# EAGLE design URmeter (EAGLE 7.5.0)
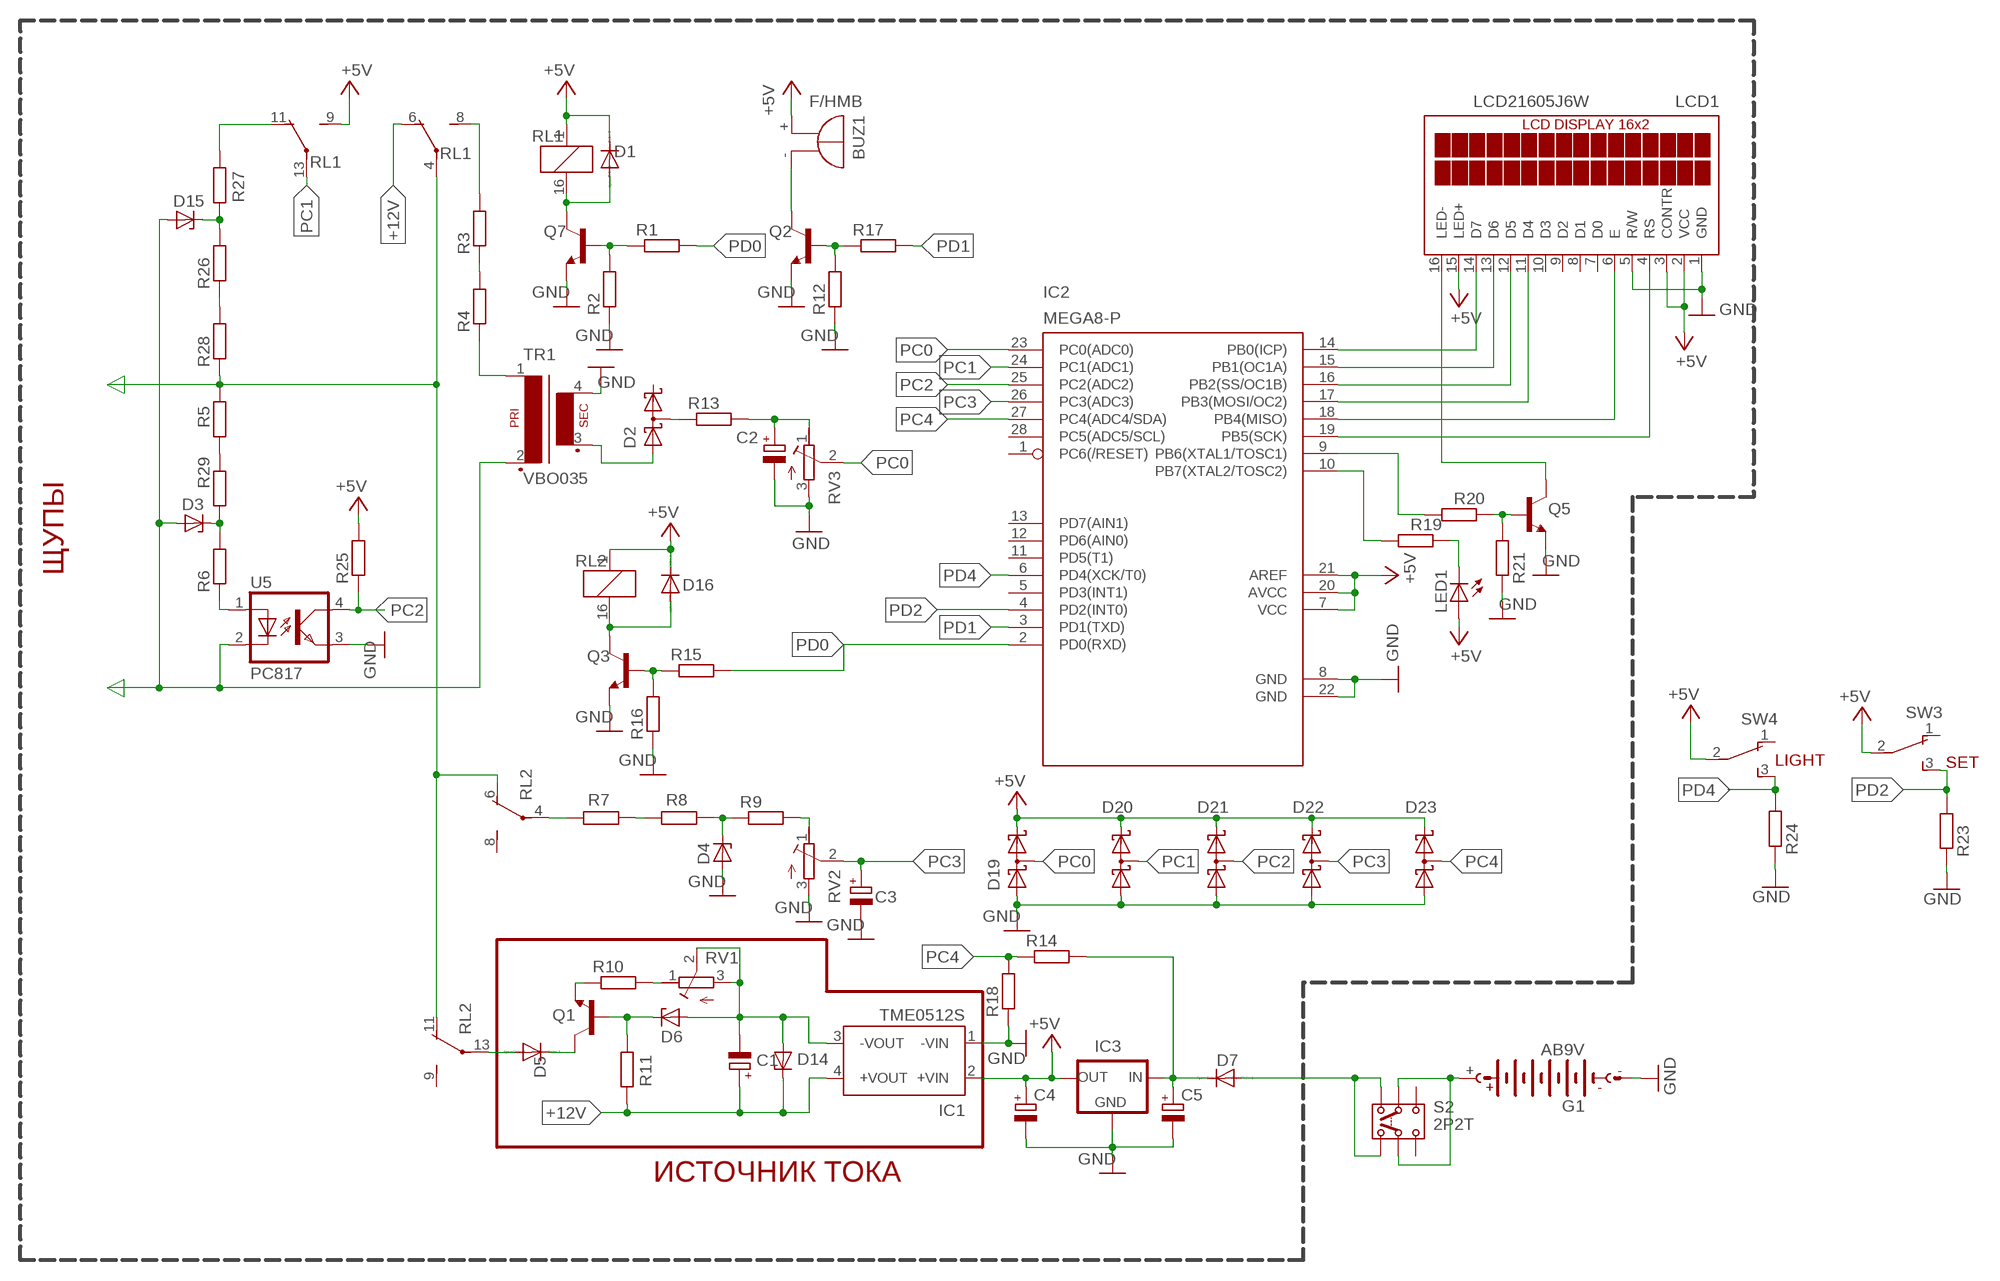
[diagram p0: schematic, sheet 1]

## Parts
BUZ1  F/HMB  [F/HMB]
C1  CPOL-EUE2-5  [E2-5]
C2  CPOL-EUE2-5  [E2-5]
C3  CPOL-EUE2-5  [E2-5]
C4  CPOL-EUE2-5  [E2-5]
C5  CPOL-EUE2-5  [E2-5]
D1  CGRM4007-G  [SOD-123_MINI-SMA]
D2  BAT54S  [SOT23]
D3  BZX85  [DO41Z10]
D4  BZX85  [DO41Z10]
D5  CGRM4007-G  [SOD-123_MINI-SMA]
D6  BZX85  [DO41Z10]
D7  CGRM4007-G  [SOD-123_MINI-SMA]
D14  BZX85  [DO41Z10]
D15  BZX85  [DO41Z10]
D16  CGRM4007-G  [SOD-123_MINI-SMA]
D19  BAT54S  [SOT23]
D20  BAT54S  [SOT23]
D21  BAT54S  [SOT23]
D22  BAT54S  [SOT23]
D23  BAT54S  [SOT23]
G1  AB9V  [AB9V]
IC1  TME0512S  [TME]
IC2  MEGA8-P  [DIL28-3]
IC3  78XXL  [78XXL]
LCD1  LCD21605J6W  [LCD21605J6W]
LED1  LED3MM  [LED3MM]
Q1  KSC5026MOS  -NPN-TO126  [TO126]
Q2  BC847  [SOT23]
Q3  BC847  [SOT23]
Q5  BC847  [SOT23]
Q7  BC847  [SOT23]
R1  R-EU_M1206  [M1206]
R2  R-EU_M1206  [M1206]
R3  R-EU_R2512  [R2512]
R4  R-EU_R2512  [R2512]
R5  R-EU_R2512  [R2512]
R6  R-EU_M1206  [M1206]
R7  R-EU_R2512  [R2512]
R8  R-EU_R2512  [R2512]
R9  R-EU_M1206  [M1206]
R10  R-EU_M1206  [M1206]
R11  R-EU_M1206  [M1206]
R12  R-EU_M1206  [M1206]
R13  R-EU_M1206  [M1206]
R14  R-EU_M1206  [M1206]
R15  R-EU_M1206  [M1206]
R16  R-EU_M1206  [M1206]
R17  R-EU_M1206  [M1206]
R18  R-EU_M1206  [M1206]
R19  R-EU_M1206  [M1206]
R20  R-EU_M1206  [M1206]
R21  R-EU_M1206  [M1206]
R23  R-EU_M1206  [M1206]
R24  R-EU_M1206  [M1206]
R25  R-EU_M1206  [M1206]
R26  R-EU_R2512  [R2512]
R27  R-EU_M1206  [M1206]
R28  R-EU_R2512  [R2512]
R29  R-EU_R2512  [R2512]
RL1  G5V-2  [G5V-2]
RL2  G5V-2  [G5V-2]
RV1  R-TRIMM-3386-F  [R-TRIMM-3386F]
RV2  R-TRIMM-3386-F  [R-TRIMM-3386F]
RV3  R-TRIMM-3386-F  [R-TRIMM-3386F]
S2  2P2T  [2P2T]
SW3  TL36WO  [TL3XWO]
SW4  TL36WO  [TL3XWO]
TR1  VBO035  [VB035]
U5  PC817  [DIL04]

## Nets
+5V: BUZ1.+ C4.+ D1.C D16.C D19.2(C2) D20.2(C2) D21.2(C2) D22.2(C2) D23.2(C2) IC1.2(+VIN) IC2.7(VCC) IC2.20(AVCC) IC2.21(AREF) IC3.OUT LCD1.2(VCC) LCD1.3(CONTR) LCD1.15(LED+) LED1.A R25.2 RL1.1 RL1.9(2:S) RL2.1 SW3.2(P) SW4.2(P)
+12V: C1.+ D14.C IC1.4(+VOUT) R11.1 RL1.6(1:O)
GND: C2.- C3.- C4.- C5.- D4.A D19.1(A1) D20.1(A1) D21.1(A1) D22.1(A1) D23.1(A1) G1.- IC1.1(-VIN) IC2.8(GND) IC2.22(GND) IC3.GND LCD1.1(GND) LCD1.5(R/W) Q2.2(E) Q3.2(E) Q5.2(E) Q7.2(E) R2.1 R12.1 R16.1 R18.1 R21.1 R23.1 R24.1 RV2.3(E) RV3.3(E) TR1.4(S4) U5.3(EMIT)
N$1: IC2.14(PB0(ICP)) LCD1.14(D7)
N$2: IC2.15(PB1(OC1A)) LCD1.13(D6)
N$3: IC2.16(PB2(SS/OC1B)) LCD1.12(D5)
N$4: IC2.17(PB3(MOSI/OC2)) LCD1.11(D4)
N$5: IC2.18(PB4(MISO)) LCD1.6(E)
N$6: IC2.19(PB5(SCK)) LCD1.4(RS)
N$7: D1.A Q7.3(C) RL1.16
N$8: Q2.1(B) R12.2 R17.1
N$9: D7.A S2.1.1 S2.1.2
N$10: Q7.1(B) R1.1 R2.2
N$11: R3.1 R4.2
N$12: R3.2 RL1.8(1:S)
N$13: R4.1 TR1.1
N$14: R5.2 R28.1 RL1.4(1:P) RL2.6(1:O) RL2.11(2:O)
N$15: D5.C Q1.2(C)
N$16: IC2.10(PB7(XTAL2/TOSC2)) R19.2
N$17: D2.1(A1) TR1.3(S3)
N$18: C2.+ R13.2 RV3.1(A)
N$19: D3.C R6.2 R29.1
N$20: R7.1 R8.2
N$21: D4.C R8.1 R9.1
N$22: R9.2 RV2.1(A)
N$23: BUZ1.- Q2.3(C)
N$24: Q3.1(B) R15.1 R16.2
N$25: D16.A Q3.3(C) RL2.16
N$26: R10.2 RV1.1(A)
N$27: D6.C Q1.3(B) R11.2
N$28: G1.+ S2.2.1 S2.2.2
N$29: C5.+ D7.C IC3.IN R14.2
N$30: R6.1 U5.1(A)
N$31: Q1.1(E) R10.1
N$32: C1.- D6.A D14.A IC1.3(-VOUT) RV1.2(S) RV1.3(E)
N$33: D15.C R26.2 R27.1
N$34: D3.A D15.A TR1.2 U5.2(C)
N$35: R7.2 RL2.4(1:P)
N$36: D5.A RL2.13(2:P)
N$37: LCD1.16(LED-) Q5.3(C)
N$38: Q5.1(B) R20.1 R21.2
N$39: IC2.9(PB6(XTAL1/TOSC1)) R20.2
N$40: D2.3(C1A2) R13.1
N$41: R26.1 R28.2
N$42: R5.1 R29.2
N$43: LED1.K(C) R19.1
PC0: D19.3(C1A2) IC2.23(PC0(ADC0)) RV3.2(S)
PC1: D20.3(C1A2) IC2.24(PC1(ADC1)) RL1.13(2:P)
PC2: D21.3(C1A2) IC2.25(PC2(ADC2)) R25.1 R27.2 RL1.11(2:O) U5.4(COL)
PC3: C3.+ D22.3(C1A2) IC2.26(PC3(ADC3)) RV2.2(S)
PC4: D23.3(C1A2) IC2.27(PC4(ADC4/SDA)) R14.1 R18.2
PD0: IC2.2(PD0(RXD)) R1.2 R15.2
PD1: IC2.3(PD1(TXD)) R17.2
PD2: IC2.4(PD2(INT0)) R23.2 SW3.3(S)
PD4: IC2.6(PD4(XCK/T0)) R24.2 SW4.3(S)
Unconnected: D2.2(C2) IC2.1(PC6(/RESET)) IC2.5(PD3(INT1)) IC2.11(PD5(T1)) IC2.12(PD6(AIN0)) IC2.13(PD7(AIN1)) IC2.28(PC5(ADC5/SCL)) LCD1.7(D0) LCD1.8(D1) LCD1.9(D2) LCD1.10(D3) RL2.8(1:S) RL2.9(2:S) S2.3.1 S2.3.2 SW3.1(O) SW4.1(O)

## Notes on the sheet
- ЩУПЫ
- LIGHT | SET
- ИСТОЧНИК ТОКА

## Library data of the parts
BUZ1 = buzzer:F/HMB: BUZZER; OC_FARNELL: unknown; OC_NEWARK: unknown
C1-C5 = rcl:CPOL-EU: POLARIZED CAPACITOR, European symbol
D1 D5 D7 D16 = diode:CGRM400*-G: Molded plasitc,JEDEC SOD-123/Mini SMA
D2 D19-D23 = diode:BAT54S: Schottky Diodes Pin connection corrected 2011-05-04 Source: Fairchild .. BAT54.pdf
D3 D4 D6 D14 D15 = diode:BZX85: Z DIODE
G1 = battery:AB9V: 9-V BATTERY CLIP
IC1 = traco-electronic:TME?*: DC/DC Converter TME Series 1 Watt Source: www.tracopower.com .. tme.pdf; MPN: TME 0512S; OC_FARNELL: 1007540; OC_NEWARK: 51R5323
IC2 = atmel:MEGA8-P: MICROCONTROLLER 8 Kbytes FLASH, 1 kbytes SRAM, 512 bytes EEPROM, USART, 4-channel 10 bit ADC, 2-channel 8 bit ADC Pin compatible with Atmega48, ATMega88, ATMega168 Source: avr.lbr; OC_FARNELL: unknown; OC_NEWARK: unknown
IC3 = v-reg:78XXL: VOLTAGE REGULATOR
LCD1 = display-lcd:LCD21605J6W
LED1 = led:LED: LED
Q1 = transistor:*-NPN-: NPN Transistror BF959 corrected 2008.03.06
Q2 Q3 Q5 Q7 = transistor:BC847: NPN TRANSISTOR
R1-R21 R23-R29 = resistor:R-EU_: RESISTOR, European symbol
RL1 RL2 = relay:G5V-2: OMRON PCB Relay Source: http://www.omron.com/ecb/products/pdf/en-g5v2.pdf; MPN: G5V-2 5DC; OC_FARNELL: 9949488; OC_NEWARK: 78K5703
RV1-RV3 = rcl:R-TRIMM-3386-F
S2 = switch:2P2T: SLIDE SWITCH 2P2T Part No. SS-22F05-G(A)4 Source: CANAL ELECTRONIC CO., LTD .. switsch.pdf
SW3 SW4 = switch:TL36WO: TINY SWITCH ON - ON Source: http://www2.produktinfo.conrad.com/datenblaetter/700000-724999/705152-da-01-de-Subminiaturschalter_TL_36WO.pdf
TR1 = trafo:VBO035
U5 = optocoupler:PC817: SHARP OPTO COUPLER; MPN: PC817X4J000F; OC_FARNELL: 9707727; OC_NEWARK: 97K7059

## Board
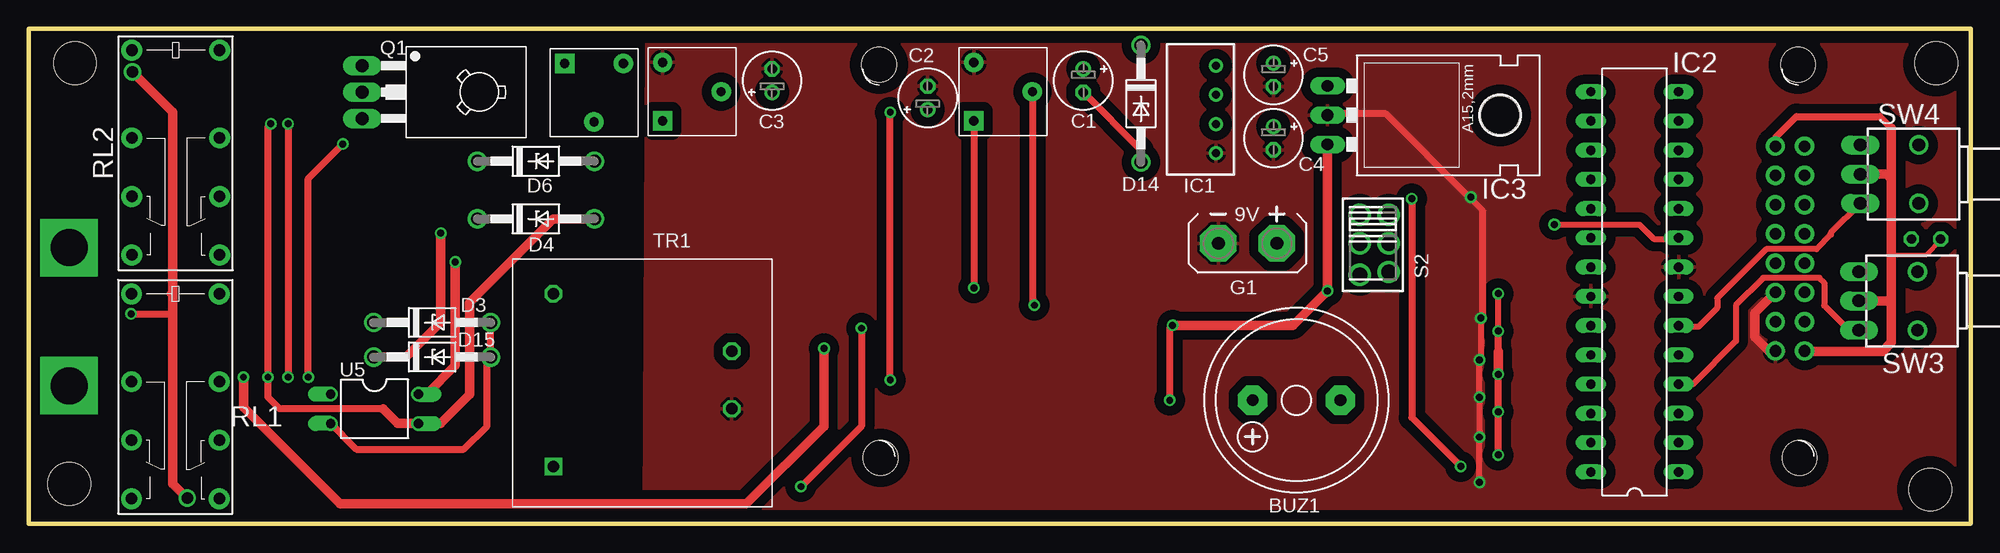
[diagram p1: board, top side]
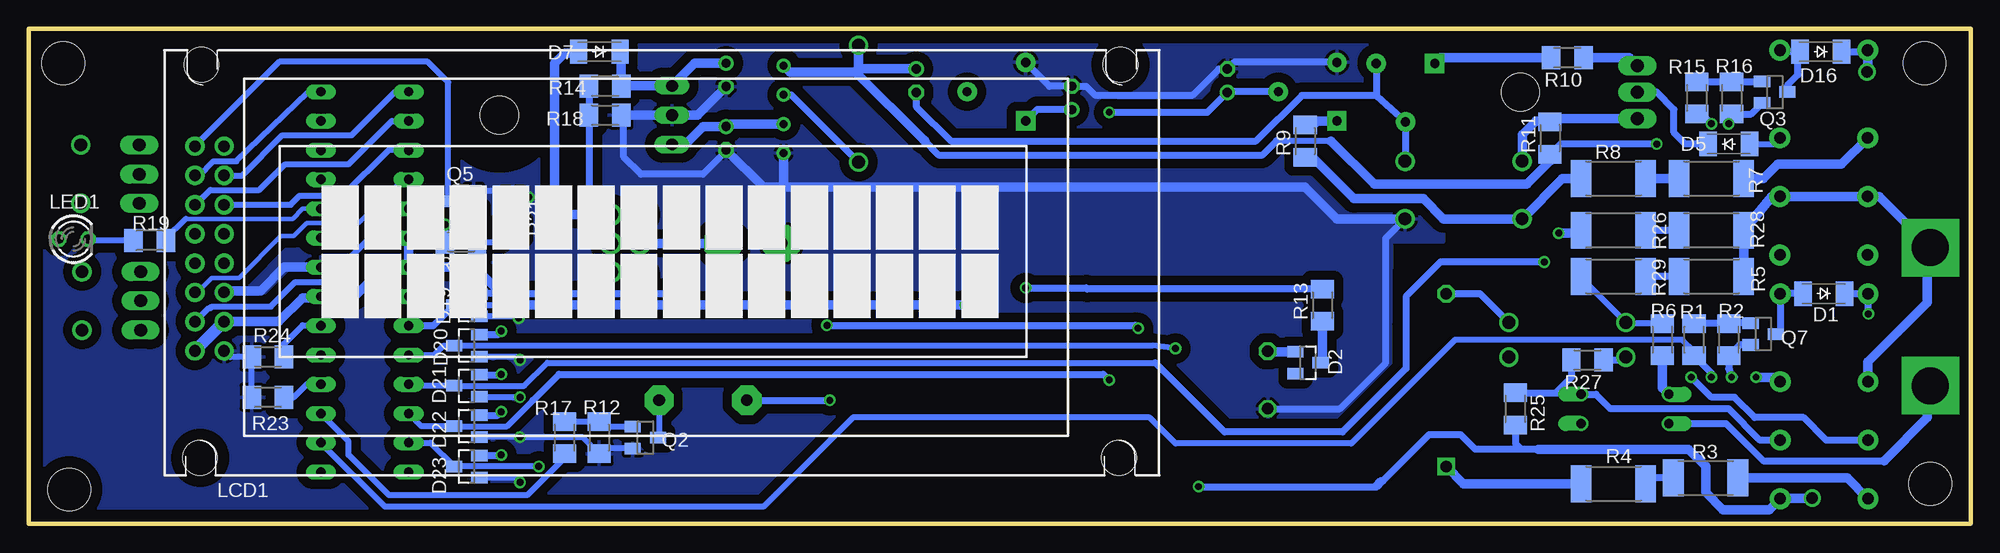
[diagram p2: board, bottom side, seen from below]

Size 168.5 x 43 mm. Coordinates in mm from the lower left corner, seen from the top.
Outline: 0,0 168.5,0 168.5,43 0,43 0,0
Copper layers (1*16): Top 0.035mm / dielectric 1.5mm / Bottom 0.035mm
Design rules "default": minimum track width 10mil, minimum drill 24mil, track to track 8mil, track to pad 8mil, pad to pad 8mil, via to via 8mil, smd to smd 8mil, copper to edge 40mil, drill to drill 8mil, minimum pad ring 10mil, minimum via ring 8mil, stop-mask expansion 4mil, vias tented up to drill 0mil, thermal gap 10mil
Holes 3.7 mm at 165.5,40 165,3 3.5,3.5 4,40

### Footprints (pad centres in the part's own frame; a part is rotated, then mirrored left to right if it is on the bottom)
F/HMB = drill 1.016 pad 2.54 octagon: + 3.81,0; - -3.81,0
E2-5 = drill 0.813 pad 1.27: + -1.016,0 | drill 0.813 pad 1.27 octagon: - 1.016,0
SOD-123_MINI-SMA = smd 1.5 x 2.1: A 1.8,0; C -1.8,0
SOT23 = smd 1 x 1.4: 1 -0.95,-1.1; 2 0.95,-1.1; 3 0,1.1
DO41Z10 = drill 1.118: A 5.08,0; C -5.08,0
AB9V = drill 1.118 pad 3.15 octagon: + 0,2.54; - 0,-2.54
TME = drill 0.7 pad 1.1: 1 -3.81,0; 2 -1.27,0; 3 1.27,0; 4 3.81,0
DIL28-3 = drill 0.813 long: 1 -16.51,-3.81; 2 -13.97,-3.81; 3 -11.43,-3.81; 4 -8.89,-3.81; 5 -6.35,-3.81; 6 -3.81,-3.81; 7 -1.27,-3.81; 8 1.27,-3.81; 9 3.81,-3.81; 10 6.35,-3.81; 11 8.89,-3.81; 12 11.43,-3.81; 13 13.97,-3.81; 14 16.51,-3.81; 15 16.51,3.81; 16 13.97,3.81; 17 11.43,3.81; 18 8.89,3.81; 19 6.35,3.81; 20 3.81,3.81; 21 1.27,3.81; 22 -1.27,3.81; 23 -3.81,3.81; 24 -6.35,3.81; 25 -8.89,3.81; 26 -11.43,3.81; 27 -13.97,3.81; 28 -16.51,3.81
78XXL = drill 1.016 long: GND 0,-3.81; IN -2.54,-3.81; OUT 2.54,-3.81 | hole 3.302: 0,11.176
LCD21605J6W = drill 1 pad 1.676: 1 2.47,-17.72; 2 -0.07,-17.72; 3 2.47,-15.18; 4 -0.07,-15.18; 5 2.47,-12.64; 6 -0.07,-12.64; 7 2.47,-10.1; 8 -0.07,-10.1; 9 2.47,-7.56; 10 -0.07,-7.56; 11 2.47,-5.02; 12 -0.07,-5.02; 13 2.47,-2.48; 14 -0.07,-2.48; 15 2.47,0.06; 16 -0.07,0.06 | hole 3: 0.375,-27; 0.5,7.125; 80.25,7.125; 80.125,-27
LED3MM = drill 0.813 octagon: A -1.27,0; K 1.27,0
TO126 = drill 1.118 long: 1 -2.286,-5.08; 2 0,-5.08; 3 2.286,-5.08 | hole 3.302: 0,5.08
M1206 = smd 1.6 x 2: 1 -1.4,0; 2 1.4,0
R2512 = smd 1.8 x 3.2: 1 -2.8,0; 2 2.8,0
G5V-2 = drill 1 pad 1.8: 1 -8.89,-3.81; 4 -1.27,-3.81; 6 3.81,-3.81; 8 8.89,-3.81; 9 8.89,3.81; 11 3.81,3.81; 13 -1.27,3.81; 16 -8.89,3.81
R-TRIMM-3386F = drill 0.8 pad 1.676 square: 1 0,0 | drill 0.8 pad 1.676: 2 5.08,2.54; 3 0,5.08
2P2T = drill 1.3 pad 1.93: 1.1 -2.492,1.38; 1.2 -2.492,-1.126; 2.1 0,1.38; 2.2 0,-1.126; 3.1 2.492,1.38; 3.2 2.746,-1.126
TL3XWO = drill 1.1 pad 1.422 long: 1 -2.54,-5.08; 2 0,-5.08; 3 2.54,-5.08 | drill 1.1 pad 1.676: M1 -2.54,0; M2 2.54,0
VB035 = drill 1 square: 1 0,0 | drill 1 octagon: 2 0,15; 3 15.5,10; 4 15.5,5
DIL04 = drill 0.813 offset: 1 -1.27,-3.81; 2 1.27,-3.81; 3 1.27,3.81; 4 -1.27,3.81

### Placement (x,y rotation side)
BUZ1  110,10.75 180 top
C1  91.5,38.5 270 top
C2  78,37 90 top
C3  64.5,38.5 90 top
C4  108,33.5 270 top
C5  108,39 270 top
D1  12.75,20 180 bottom
D2  57.5,14 270 bottom
D3  35,17.5 0 top
D4  44,26.5 0 top
D5  21,33 0 bottom
D6  44,31.5 0 top
D7  119,41 180 bottom
D14  96.5,36.5 270 top
D15  35,14.5 0 top
D16  13,41 180 bottom
D19  130.5,19 90 bottom
D20  130.5,15.5 90 bottom
D21  130.5,12 90 bottom
D22  130.5,8.5 90 bottom
D23  130.5,5 90 bottom
G1  105.75,24.38 270 top
IC1  103,36 90 top
IC2  139.35,21.03 90 top
IC3  116.5,35.5 270 top
LCD1  154.02,32.75 0 bottom
LED1  164.62,24.75 0 bottom
Q1  34,37.5 270 top
Q2  115,7.5 270 bottom
Q3  17,37.5 270 bottom
Q5  131,28 90 bottom
Q7  18,16.5 270 bottom
R1  24,16 270 bottom
R2  21,16 90 bottom
R3  23,4 0 bottom
R4  31,3.5 0 bottom
R5  22.5,21.5 0 bottom
R6  26.75,16 90 bottom
R7  22.5,30 0 bottom
R8  31,30 0 bottom
R9  57.75,33.25 90 bottom
R10  35,40.5 180 bottom
R11  36.5,33.5 90 bottom
R12  119,7.5 90 bottom
R13  56.25,19 90 bottom
R14  118.5,38 0 bottom
R15  23.75,37 270 bottom
R16  20.75,37 90 bottom
R17  122,7.5 270 bottom
R18  118.5,35.5 180 bottom
R19  158,24.62 0 bottom
R20  131,24.5 180 bottom
R21  126.5,27 270 bottom
R23  147.75,11 0 bottom
R24  147.75,14.5 0 bottom
R25  39.5,10 270 bottom
R26  31,25.5 180 bottom
R27  33.25,14.25 180 bottom
R28  22.5,25.5 180 bottom
R29  31,21.5 0 bottom
RL1  12.72,11.09 270 top
RL2  12.75,32.25 270 top
RV1  46.5,40 270 top
RV2  55,35 0 top
RV3  82,35 0 top
S2  116.62,24.38 270 top
SW3  163.88,19.38 270 top
SW4  164,30.38 270 top
TR1  45.5,5 0 top
U5  30,10 270 top

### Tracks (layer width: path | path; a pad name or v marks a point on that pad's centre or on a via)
+5V  (via drill 0.6, 1)
  Top 0.406: LED1.A 165.9,24.64 164.62,23.38 161.62,23.38
  Top 0.51: v127.5,16.75 v127.5,20
  Top 0.61: 127.5,15 v127.5,16.75 | v127.5,13 v127.5,9.75 v127.5,6 | 12.25,20 12.5,19.75 | v99,10.75 99,17 v99.25,17.25 | v72.25,17 72.25,8.5 v67,3.25 | LCD1.15 151.55,33.55 153.38,35.38 160.62,35.38 161.62,34.38 | v8.88,18.25 12.38,18.25 12.5,18.38
  Top 0.813: v9,39.25 12.5,35.75 12.5,19.75 12.5,18.38 12.5,3.5 v13.75,2.25 | v127.5,13 127.5,15 | IC3.OUT v112.69,20.25 109.69,17.25 v99.25,17.25 | LCD1.2 154.12,15 160.88,15 161.62,15.75 161.62,19.25 | 161.62,34.38 161.62,30 | 161.62,30 161.62,23.38 161.62,19.25 | SW3.2 161.5,19.38 161.62,19.25 | SW4.2 161.25,30.38 161.62,30
  Bottom 0.61: D21.2 127.55,12.95 v127.5,13 | D19.2 129.35,20 v127.5,20 112.94,20 v112.69,20.25 | D20.2 127.8,16.45 v127.5,16.75 | D22.2 127.8,9.45 v127.5,9.75 | D23.2 127.55,5.95 v127.5,6 | 37.5,6.5 39,6.5 | 39,6.5 43,6.5 44.25,7.75 47,7.75 51,3.75 | 51,3.75 51.25,3.75 51.75,3.25 | BUZ1.+ v99,10.75 | v99.25,17.25 72.5,17.25 v72.25,17 | v67,3.25 51.5,3.25 51,3.75 | 39.5,8.5 39.5,7 39,6.5 | D16.C 9.08,41 RL2.1 | v8.88,18.25 8.91,18.29 RL1.1 8.93,20 D1.C
  Bottom 0.813: RL2.1 8.94,39.31 v9,39.25 | v13.75,2.25 16.48,2.25 RL1.9 17.48,1.25 21.5,1.25 23,2.75 23,5 24.5,6.5 37.5,6.5 | R25.2 39.5,8.5 | IC1.2 107.79,34.73 C4.+ 109.98,34.52 111.5,33 112.65,33 IC3.OUT | LCD1.3 146.81,17.57 144.75,19.62 143.29,19.62 IC2.7 140.24,19.76 137.75,22.25 135.59,22.25 IC2.21 | IC2.20 IC2.21 | IC2.21 129.8,22.3 v127.5,20
  Bottom 1.016: LCD1.3 LCD1.2
+12V  (via drill 0.6)
  Top 0.61: v24.25,12.75 24.25,30 v27.25,33
  Bottom 0.51: 55.5,33.25 60.25,33.25
  Bottom 0.61: RL1.6 12.53,7.28 14.5,9.25 18.75,9.25 20.5,11 22.5,11 v24.25,12.75 | v27.25,33 35.6,33 R11.1 | 60.25,33.25 61.5,32 89.5,32 90.88,33.38
  Bottom 0.813: R11.1 36.5,31.5 38.5,29.5 51.75,29.5 55.5,33.25 | 90.75,33.25 90.88,33.38 96.75,39.25 | 96.75,39.25 102.44,39.25 IC1.4 | C1.+ 96.48,39.52 | 96.48,39.52 96.75,39.25 | D14.C 96.5,39.53 96.48,39.52
GND  (via drill 0.6)
  Top 0.51: v125.88,3.62 v125.88,7.55 v125.88,11 v125.88,14.25 126,14.38 v126,17.88 | v125.12,28.38 125.12,28.25 126.12,27.25
  Top 0.61: 30.75,10 21.75,10 20.75,11 v20.75,12.75 20.75,34.5 v21,34.75 | 126.12,27.25 126.12,18 v126,17.88 | v125.15,28.4 124.97,28.4 117.75,35.62 112.81,35.62 IC3.GND
  Top 0.813: 30.75,10 32.02,8.73 U5.3 35.73,8.73 38.25,11.25 38.25,19.25 45.5,26.5 D4.A | LCD1.1 150.97,15.03 149.75,16.25 149.75,18.31 LCD1.5
  Bottom 0.51: Q2.2 118.55,6.55 R12.1 120.45,7.55 v125.88,7.55 D22.1 | Q5.2 127.05,28.95 R21.1 v125.15,28.4 v125.12,28.38 | R23.1 R24.1 151.02,14.5 LCD1.1 | D23.1 126.3,4.05 v125.88,3.62 | D20.1 126.17,14.55 v125.88,14.25 | D21.1 125.92,11.05 v125.88,11 | D19.1 126.17,18.05 v126,17.88
  Bottom 0.61: Q3.2 19.05,35.6 R16.1 21,35.35 v21,34.75 | Q7.2 20.05,15.55 R2.1 21,13.5 v20.75,12.75 20.5,12.75 | TR1.4 54.75,10 50.75,14 50.75,24.83 D4.A | RV2.3 63.94,40.08 C3.- 64.52,39.5 65.25,39.5 67.5,37.25 76,37.25 76.77,38.02 C2.- 79.94,38.02 RV3.3 | C4.- 108,32.38 110,30.38 115.38,30.38 116.88,31.88 116.88,35.27 R18.1
  Bottom 0.813: D4.A 55,26.5 57.75,29.25 103,29.25 | 103,29.25 104.77,29.25 C4.- | IC1.1 103,29.25 | C5.- 110.48,35.5 IC3.GND R18.1 | IC2.8 146.32,22.3 148.38,20.25 151.41,20.25 LCD1.5 | G1.- 103.21,29.04 103,29.25
  pour Top (isolate 0.813): 53.62,42 53.38,0.88 168,0.88 168,42.12
  pour Bottom (isolate 0.813): 47.88,41.88 45.75,41.88 45.75,24.5 50.25,24.5 50.5,1 167.75,0.75 167.75,41.88
N$1
  Bottom 0.51: LCD1.14 153.73,30.27 152.5,31.5 150.5,31.5 144.25,37.5 143.2,37.5 IC2.14
N$2
  Bottom 0.51: LCD1.13 149.98,30.27 146.5,33.75 140.5,33.75 136.75,37.5 135.58,37.5 IC2.15
N$3
  Bottom 0.51: LCD1.12 154.02,27.73 152.75,29 148.5,29 146.25,31.25 140.75,31.25 137,35 IC2.16
N$4
  Bottom 0.51: LCD1.11 145.77,27.73 145,28.5 141.25,28.5 137.25,32.5 135.58,32.5 IC2.17
N$5
  Bottom 0.406: LCD1.6 153.89,20.11 152.62,21.38 150.25,21.38 146.62,25 145.5,25 144.38,26.12 139.88,26.12 136.12,29.88 135.59,29.88 IC2.18
N$6
  Bottom 0.51: LCD1.4 154.06,17.57 152.88,18.75 152.75,18.75 152.62,18.88 147.5,18.88 145.38,21 141.5,21 140.62,21.88 140.62,23.12 136.38,27.38 IC2.19
N$7
  Bottom 0.61: D1.A 16.51,20 RL1.16 16.53,16.87 Q7.3
N$8
  Bottom 0.51: R17.1 R12.2 118.55,8.45 Q2.1
N$9
  Bottom 0.813: D7.A 120.92,40.88 122,40.88 122.88,40 122.88,27.75 121.99,26.87 S2.1.1 S2.1.2
N$10
  Bottom 0.61: Q7.1 20.95,17.45 R2.2 R1.1
N$11
  Bottom 0.61: R3.1 27.7,4 R4.2
N$12
  Bottom 0.813: R3.2 10.71,4 RL1.8
N$13
  Bottom 0.813: R4.1 44,3.5 TR1.1
N$14  (via drill 3.2 pad 5)
  Bottom 0.813: R5.2 R28.1 17.26,28.44 RL2.11 RL2.6 7.94,28.44 v3.5,24 3.75,23.75 3.75,19.25 8.91,14.09 RL1.4
N$15
  Bottom 0.61: D5.C 24.75,33 25.75,34 25.75,36 27.25,37.5 Q1.2
N$16
  Bottom 0.406: R19.2 156.6,24.77 | 154.88,26.5 145.62,26.5 144.75,27.38 IC2.10
  Bottom 0.5: 156.6,24.77 154.88,26.5
N$17
  Bottom 0.813: D2.1 60.95,14.95 TR1.3
N$18  (via drill 0.6)
  Top 0.61: RV3.1 v82,20.5
  Bottom 0.61: R13.2 76.65,20.4 76.75,20.5 v82,20.5 | C2.+ 81.02,35.98 RV3.1
N$19
  Bottom 0.51: R6.2 29.82,17.4 D3.C 33.42,21 R29.1
N$20
  Bottom 0.813: R7.1 R8.2
N$21
  Bottom 0.813: R9.1 57.1,31.85 53.5,28.25 47.5,28.25 45.75,26.5 D4.C 35.42,30 R8.1
N$22
  Bottom 0.813: RV2.1 56.75,35 57.25,34.5 57.6,34.5 R9.2
N$23
  Bottom 0.51: BUZ1.- 113.81,7.59 Q2.3
N$24
  Bottom 0.61: Q3.1 18.15,38.4 R16.2 R15.1
N$25
  Bottom 0.61: Q3.3 15.9,38.1 15,39 15,40.8 D16.A 16.42,41 RL2.16
N$26
  Bottom 0.813: R10.2 46,40.5 RV1.1
N$27
  Bottom 0.813: Q1.3 36.19,35.21 R11.2 36.6,35 37.75,35 38.92,33.83 D6.C
N$28
  Bottom 0.813: G1.+ S2.2.2 S2.2.1
N$29
  Bottom 0.813: C5.+ 110.71,40.02 IC3.IN 117.06,38.04 R14.2 117.1,40.4 D7.C
N$30
  Bottom 0.813: R6.1 26.75,11.83 U5.1
N$31
  Bottom 0.813: R10.1 29.63,40.5 Q1.1
N$32
  Top 0.61: D14.A 96.5,32.48 C1.-
  Bottom 0.61: D6.A 49.04,32.54 RV1.2 51.58,37.21 | RV1.3 51.58,37.21 | 51.58,37.21 58.04,37.21 62,33.25 88.5,33.25 91.5,36.25 C1.- | IC1.3 102.35,37.27 D14.A
N$33  (via drill 0.6)
  Top 0.813: D15.C 32.75,14.5 35.75,17.5 v35.75,25.25
  Bottom 0.61: R27.1 30.17,14.25 D15.C
  Bottom 0.813: 30,14.42 D15.C | v35.75,25.25 34.05,25.25 R26.2
N$34  (via drill 3.2 pad 5)
  Top 0.61: D3.A D15.A 39.75,14.17 39.75,8.5 37.75,6.5 28.42,6.5 U5.2
  Bottom 0.61: TR1.2 42.58,20 D3.A | U5.2 21.23,8.73 18,5.5 7.5,5.5
  Bottom 0.813: 7.5,5.5 3.75,9.25 3.75,11.75 v3.5,12
N$35
  Bottom 0.813: R7.2 18,30 16.75,31.25 11.21,31.25 RL2.4
N$36
  Bottom 0.51: D5.A 17.08,33 RL2.13
N$37
  Bottom 0.51: Q5.3 132.1,38.35 133.88,40.12 146.78,40.12 LCD1.16
N$38
  Bottom 0.51: R21.2 127.6,24.5 R20.1 129.9,24.8 Q5.1
N$39  (via drill 0.6)
  Top 0.51: v132.38,26 139.75,26 141,24.75 143.07,24.75 IC2.9
  Bottom 0.51: R20.2 132.4,25.98 v132.38,26
N$40
  Bottom 0.813: R13.1 56.25,14.15 D2.3
N$41
  Bottom 0.61: R28.2 R26.1
N$42
  Bottom 0.61: R5.1 R29.2
N$43
  Bottom 0.406: 163.35,24.62 LED1.K
  Bottom 0.5: R19.1 163.35,24.62
PC0  (via drill 0.6)
  Top 0.61: RV3.2 87.08,19.17 v87.25,19
  Bottom 0.51: D19.3 126.25,19
  Bottom 0.61: IC2.23 133.38,17.22 D19.3
  Bottom 0.813: 126.25,19 89.5,19 v87.25,19
PC1  (via drill 0.6)
  Top 0.813: v69,15.25 69,8.5 62.25,1.75 27,1.75 18.62,10.12 v18.62,12.75
  Bottom 0.51: IC2.24 133.32,14.68 132.5,15.5 D20.3 71,15.5 v69,15.25
  Bottom 0.813: v18.62,12.75 16.92,12.75 RL1.13
PC2  (via drill 0.6)
  Top 0.813: U5.4 34.52,11.27 37,13.75 v37,22.75
  Bottom 0.51: IC2.25 135.4,12 D21.3 125.5,12 123.5,14 70.75,14
  Bottom 0.61: v37,22.75 46,22.75 49,19.75 49,13.5 54.5,8 64.75,8 70.75,14 | R25.1 36,11.4 | 36,11.4 33.94,11.4 U5.4 32.52,11.27 31.25,10 21,10 18.28,7.28 RL1.11 | R27.2 34.65,12.75 36,11.4
PC3  (via drill 0.6)
  Top 0.61: v74.75,12.5 v74.75,35.75
  Bottom 0.51: IC2.26 134.44,8.5 D22.3 127,8.5 124.75,10.75
  Bottom 0.61: 124.75,10.75 122.5,13 75.25,13 v74.75,12.5 | v74.75,35.75 66.23,35.75 C3.+ 64.44,37.54 RV2.2
PC4  (via drill 0.6)
  Top 0.61: v120,28.25 120,9.25 v124.25,5
  Bottom 0.51: v124.25,5 D23.3 133.66,7.06 IC2.27
  Bottom 0.61: R14.1 R18.2 119.9,28.35 v120,28.25
PD0  (via drill 0.6)
  Top 0.61: v22.5,34.75 v22.5,12.75
  Bottom 0.51: R1.2 24,15 25,16 44.75,16 53.75,7 69,7 71.25,9.25 97,9.25 104.75,1.5 137.6,1.5 IC2.2
  Bottom 0.61: R15.2 23.35,35.6 v22.5,34.75 | v22.5,12.75 22.5,13.1 R1.2
PD1
  Bottom 0.51: R17.2 122,5.75 125.25,2.5 137.25,2.5 140.75,6 140.75,7.19 IC2.3
PD2
  Top 0.51: IC2.4 143.18,12.12 144.38,12.12 148.12,15.88 148.12,19 150.5,21.38 155.38,21.38 155.79,20.96 155.79,18.96 157.88,16.88 158.75,16.88 SW3.3
  Bottom 0.51: R23.2 145.5,11 144.38,12.12 143.18,12.12 IC2.4
PD4
  Top 0.51: IC2.6 143.25,17.12 144.88,17.12 146.5,18.75 146.5,19.62 150.75,23.88 155.12,23.88 156.38,25.12 156.38,25.29 SW4.3
  Bottom 0.51: R24.2 146.35,15.65 144.75,17.25 143.19,17.25 IC2.6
